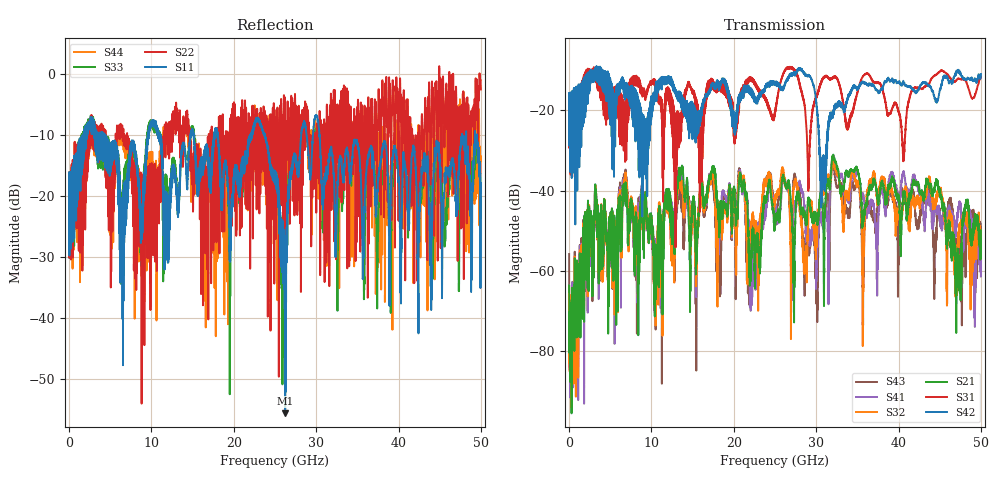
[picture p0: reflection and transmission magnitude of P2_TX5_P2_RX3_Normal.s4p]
!Keysight Technologies,N5225B,MY57041031,A.13.20.10
!Date: Friday, May 31, 2019 11:31:08
!Correction: S11(Full 4 Port(1,2,3,4))
!S12(Full 4 Port(1,2,3,4))
!S13(Full 4 Port(1,2,3,4))
!S14(Full 4 Port(1,2,3,4))
!S21(Full 4 Port(1,2,3,4))
!S22(Full 4 Port(1,2,3,4))
!S23(Full 4 Port(1,2,3,4))
!S24(Full 4 Port(1,2,3,4))
!S31(Full 4 Port(1,2,3,4))
!S32(Full 4 Port(1,2,3,4))
!S33(Full 4 Port(1,2,3,4))
!S34(Full 4 Port(1,2,3,4))
!S41(Full 4 Port(1,2,3,4))
!S42(Full 4 Port(1,2,3,4))
!S43(Full 4 Port(1,2,3,4))
!S44(Full 4 Port(1,2,3,4))
!S4P File: Measurements: <S11,S12,S13,S14>,
!<S21,S22,S23,S24>,
!<S31,S32,S33,S34>,
!<S41,S42,S43,S44>:
# Hz S  dB  R 50.0
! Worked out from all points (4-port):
!   5000 points, 10 MHz to 50 GHz, reference 50 ohm
!   strongest paths, dB at 10 MHz, 12.51 GHz, 25.01 GHz, 37.51 GHz, 50 GHz:
!     S42: -19.4, -14.1, -13.2, -15.2, -11.0
!     S31: -19.5, -17.8, -20.9, -13.1, -11.7
!     S21: -63.7, -46.8, -48.4, -42.5, -49.9
!     S32: -63.8, -47.8, -42.2, -42.6, -49.9
!     S41: -70.0, -45.6, -44.5, -50.0, -61.4
!     S43: -55.8, -46.1, -44.7, -43.5, -49.8
!   lowest |S11| = -55.6 dB at 26.24 GHz (marker M1), VSWR 1.00, Z = 49.9 + j0.145 ohm
!   |S11| at or under -10 dB: 4.282 GHz to 9.568 GHz (5.286 GHz wide, 76.3 % of centre); 23.74 GHz to 28.18 GHz (4.44 GHz wide, 17.1 % of centre); 30.41 GHz to 47.7 GHz (17.29 GHz wide, 44.3 % of centre)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
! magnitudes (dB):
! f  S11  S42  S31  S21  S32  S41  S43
! 10 MHz  -19.9  -19.4  -19.5  -63.7  -63.8  -70.0  -55.8
! 3.29 GHz  -12.9  -9.4  -12.9  -40.7  -40.7  -41.4  -41.4
! 20.77 GHz  -16.3  -17.6  -16.1  -35.5  -36.1  -34.9  -35.7
! 22.2 GHz  -9.9  -16.2  -12.6  -55.3  -47.7  -62.9  -50.5
! 26.24 GHz  -55.6  -13.5  -9.9  -38.3  -38.6  -37.2  -38.1
! 30.78 GHz  -21.4  -33.2  -12.3  -43.6  -40.5  -48.2  -44.0
! 50 GHz  -19.5  -11.0  -11.7  -49.9  -49.9  -61.4  -49.8
